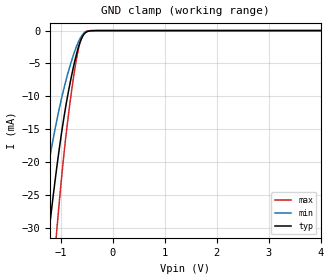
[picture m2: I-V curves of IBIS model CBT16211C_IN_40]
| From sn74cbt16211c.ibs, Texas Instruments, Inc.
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[Model]   CBT16211C_IN_40
Model_type  Input
Vinl=0.8
Vinh=2.0
| variable   typ   min   max
C_comp   3.93pF   2.55pF   6.70pF
[Temperature Range]   40   100   -40
| Ambient temperature   25   85   -40
[Voltage range]   4   4   4
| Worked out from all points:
|   GND clamp passes 1 mA (typ) near -0.59 V on its own axis
[GND Clamp]
| CBT16211C_IN_40
|   Voltage   I(typ)   I(min)   I(max)
-4V       -307.6mA   -226.2mA   -397.9mA
-1.435V   -46.42mA   -30.48mA   -67.92mA
-1.24V    -31.69mA   -20.74mA   -46.67mA
-1.205V   -29.25mA   -19.14mA   -43.07mA
-1.08V    -21.14mA   -13.89mA   -30.9mA
-910mV    -11.91mA   -7.942mA   -16.81mA
-755mV    -5.562mA   -3.735mA   -7.234mA
-695mV    -3.56mA    -2.396mA   -4.286mA
-635mV    -1.944mA   -1.323mA   -2.02mA
-580mV    -909.9uA   -647.5uA   -742.7uA
-515mV    -268.8uA   -219.5uA   -144.4uA
4V        162.4pA    581.9pA    36.11pA
